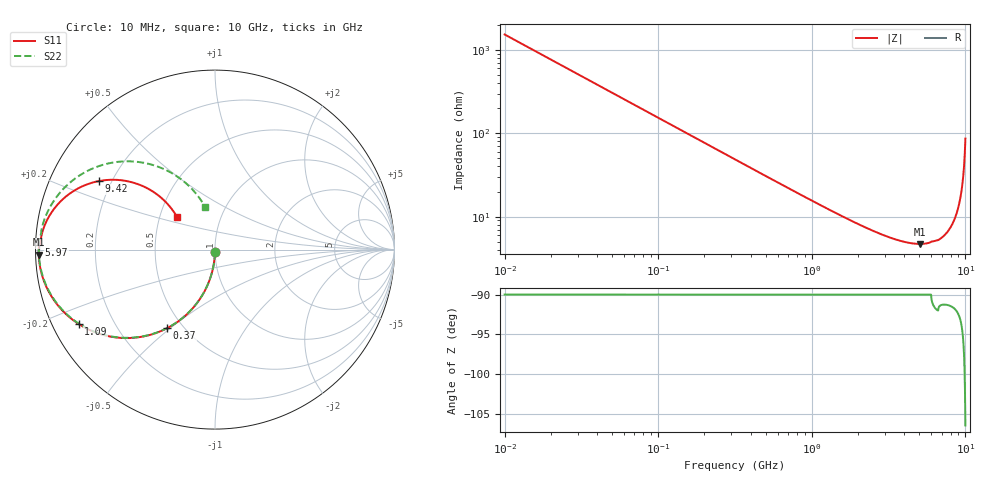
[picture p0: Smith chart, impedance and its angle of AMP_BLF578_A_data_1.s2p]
! Created Mon Oct  5 17:39:55 2009
# ghz S ma R 50
! 2 Port Network Data from SP1.SP block
! freq  magS11  angS11  magS21  angS21  magS12  angS12  magS22  angS22
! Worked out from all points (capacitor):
!   1000 points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, 10 MHz to 10 GHz, reference 50 ohm
!   read as one part in shunt: C = 10.4 pF near 60 MHz
!   lowest |Z| = 4.71 ohm at 5.06 GHz (marker M1)
!   S11 on the Smith chart (normalised r, x): 10 MHz: 1.00, -0.03; 370 MHz: 0.41, -0.49; 1.09 GHz: 0.08, -0.25; 5.97 GHz: 0.01, +0.01; 9.42 GHz: 0.15, +0.27; 10 GHz: 0.62, +0.24
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0.01  0.01615 -90.9  0.9999 -0.9  0.9999 -0.9  0.01615 -90.9
0.08  0.1282 -97.5  0.9917 -7.5  0.9917 -7.5  0.1282 -97.5
0.13  0.2055 -102.0  0.9787 -12.0  0.9787 -12.0  0.2055 -102.1
0.23  0.3481 -110.7  0.9375 -20.7  0.9375 -20.7  0.3481 -110.7
0.37  0.5123 -121.3  0.8588 -31.4  0.8588 -31.4  0.5123 -121.4
0.52  0.6417 -130.6  0.767 -40.7  0.767 -40.7  0.6417 -130.7
0.72  0.7557 -140.0  0.6548 -50.1  0.6548 -50.1  0.7557 -140.2
1.09  0.8657 -151.4  0.5006 -61.6  0.5006 -61.6  0.8657 -151.7
1.68  0.9333 -161.3  0.3591 -71.5  0.3591 -71.5  0.9333 -161.7
2.45  0.9636 -168.0  0.2674 -78.3  0.2674 -78.3  0.9636 -168.7
3.34  0.9763 -172.6  0.2163 -83.1  0.2163 -83.1  0.9763 -173.5
5.01  0.9824 -178.2  0.1866 -89.0  0.1866 -89.0  0.9824 -179.8
5.06  0.9824 -178.4  0.1866 -89.2  0.1866 -89.2  0.9824 180.0
5.97  0.9804 178.6  0.1969 -92.4  0.1969 -92.4  0.9803 176.6
6.67  0.9709 176.7  0.2059 -96.4  0.2059 -96.4  0.9731 174.2
8.34  0.9354 167.4  0.3257 -106.6  0.3257 -106.6  0.9366 162.8
8.97  0.8739 159.6  0.4496 -116.1  0.4496 -116.1  0.8745 153.1
9.42  0.7527 149.6  0.6107 -129.1  0.6107 -129.1  0.751 139.9
9.61  0.6518 143.6  0.7044 -137.8  0.7044 -137.8  0.647 131.0
9.76  0.5359 138.7  0.785 -146.6  0.785 -146.6  0.5261 122.0
9.87  0.4268 136.2  0.8416 -154.4  0.8416 -154.4  0.4097 114.0
10  0.2781 139.4  0.8948 -164.8  0.8948 -164.8  0.2408 102.8
